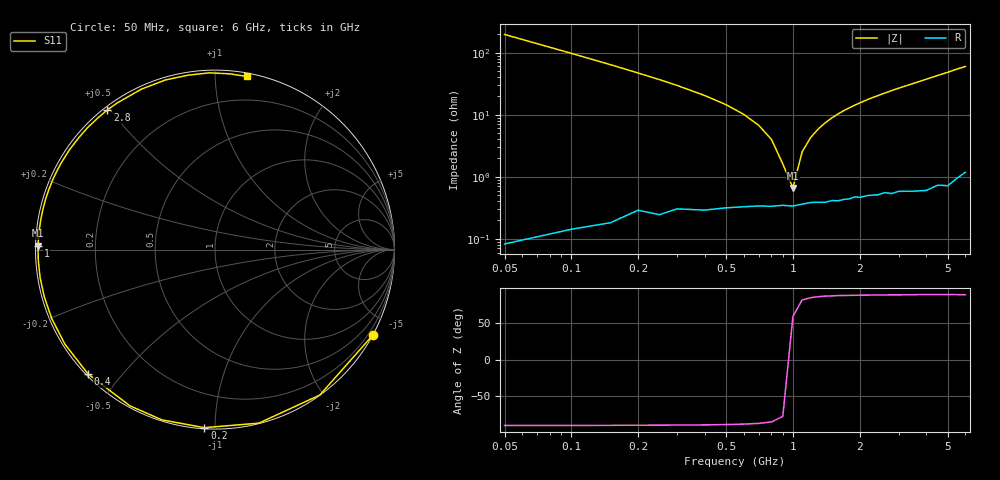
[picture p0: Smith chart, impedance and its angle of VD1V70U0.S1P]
! Infineon Technologies  Discrete & RF Semiconductors
! BBY 55-03
! Si Tuning Diode in SOD323
! VR = 1.75 V
! S-Parameters:  June  1999
# GHz  S  MA  R  50
!  f  S11
! GHz  MAG  ANG
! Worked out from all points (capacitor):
!   34 points, 50 MHz to 6 GHz, reference 50 ohm
!   read as one part to ground: C = 16.1 pF near 50 MHz
!   lowest |Z| = 660 mohm at 1 GHz (marker M1)
!   series resonance near 973.5 MHz, so ESL is about 1.7 nH
!   S11 on the Smith chart (normalised r, x): 50 MHz: 0.00, -3.94; 200 MHz: 0.01, -0.94; 400 MHz: 0.01, -0.41; 1 GHz: 0.01, +0.01; 2.8 GHz: 0.01, +0.49; 6 GHz: 0.02, +1.20
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0.05  0.9998 -28.5
0.1  0.9988 -54.2
0.15  0.9973 -75.8
0.2  0.9939 -93.4
0.25  0.9937 -107.3
0.3  0.9911 -118.6
0.4  0.9901 -135.6
0.5  0.9884 -147.7
0.6  0.9875 -157.1
0.7  0.9868 -164.6
0.8  0.9868 -170.9
0.9  0.9863 -176.4
1  0.9866 178.7
1.1  0.9857 174.3
1.3  0.9848 166.6
1.6  0.9844 156.7
1.8  0.9837 150.9
2  0.9831 145.6
2.2  0.9824 140.6
2.4  0.9827 136.1
2.8  0.9829 127.6
3  0.9821 123.7
3.5  0.9835 114.7
4  0.9847 106.3
4.5  0.9833 98.7
5  0.9853 91.8
5.5  0.9828 85.2
6  0.9809 79.5
